[IBIS Ver]   5.0
[Comment Char] |_char
[File name]   k61_120_143wlcsp_full.ibs
[File Rev]   1.1
[Date]   November 08,2016
[Source]   Cadence SpeedXP Suite XtractIM 13.0.2.01241
[Notes]   IBIS model for K61 microprocessor covers 1.71 - 3.6V range
[Disclaimer]   The model given below represents 143WLCSP package on K61 family.
[Copyright]   Copyright, NXP Semiconductors, 2016
|  Component K61
[Component]   K61
[Manufacturer]  NXP Semiconductors
[Package]
|   typ   min   max
R_pkg   0.30362   0.061464   1.7211
L_pkg   1.444e-9   5.12e-10   8.838e-9
C_pkg   1.994e-13   4.495e-14   3.303e-13
[Pin]   Signal_name   model_name   R_pin   L_pin   C_pin
L8   VBAT   POWER
C4   VDD   POWER
E5   VDD   POWER
E7   VDD   POWER
F7   VDD   POWER
G5   VDD   POWER
G7   VDD   POWER
K2   VDD   POWER
L2   VDD   POWER
K11   VDDA   POWER
G9   VOUT33   POWER
K10   VREFH   NC
K9   VREFL   NC
J7   VREFOUT   NC
G8   VREGIN   POWER
L11   DAC0OUT   NC   0.24254   1.143e-9   1.779e-13
K7   DAC1OUT   NC   0.50782   2.109e-9   3.009e-13
L9   EXTAL32   NC   1.7211   8.838e-9   5.089e-14
J10   PGA0DM   NC   0.30343   1.365e-9   2.136e-13
J11   PGA0DP   NC   0.2527   1.165e-9   1.937e-13
J8   PGA1DM   NC   0.42945   1.888e-9   2.645e-13
J9   PGA1DP   NC   0.36354   1.605e-9   2.699e-13
H10   PGA2DM   NC   0.30536   1.372e-9   2.422e-13
H11   PGA2DP   NC   0.23989   1.123e-9   1.938e-13
H8   PGA3DM   NC   0.43162   1.879e-9   2.993e-13
H9   PGA3DP   NC   0.36665   1.611e-9   2.843e-13
K6   PTA0   io_5vtol   0.28835   1.325e-9   2.168e-13
J6   PTA1   io_5vtol   0.3552   1.577e-9   2.756e-13
H5   PTA2   io_5vtol   0.41339   1.804e-9   3.263e-13
J5   PTA3   io_5vtol   0.34455   1.522e-9   2.833e-13
K5   PTA4   io_5vtol   0.28456   1.277e-9   2.245e-13
L5   PTA5   io_5vtol   0.23851   1.144e-9   1.725e-13
L4   PTA12   io_fast_5vtol   0.15229   7.498e-10   1.465e-13
K4   PTA13   io_fast_5vtol   0.21258   9.941e-10   1.823e-13
J4   PTA14   io_fast_5vtol   0.27735   1.255e-9   2.014e-13
L3   PTA15   io_fast_5vtol   0.15747   7.655e-10   1.477e-13
K3   PTA16   io_fast_5vtol   0.22512   1.035e-9   1.845e-13
J3   PTA17   io_fast_5vtol   0.29053   1.305e-9   2.042e-13
L1   PTA18   io_5vtol   0.16163   9.058e-10   5.625e-14
K1   PTA19   io_5vtol   0.14133   7.969e-10   8.082e-14
H4   PTB0   io_5vtol   0.35239   1.586e-9   2.293e-13
H3   PTB1   io_5vtol   0.28722   1.315e-9   2.234e-13
H2   PTB2   io_5vtol   0.22237   1.056e-9   1.795e-13
H1   PTB3   io_5vtol   0.15814   8.112e-10   1.487e-13
G4   PTB4   io_5vtol   0.35452   1.598e-9   2.246e-13
G3   PTB5   io_5vtol   0.28978   1.342e-9   2.086e-13
G2   PTB6   io_5vtol   0.22499   1.085e-9   1.769e-13
G1   PTB7   io_5vtol   0.16003   8.338e-10   1.531e-13
F4   PTB8   io_5vtol   0.35932   1.606e-9   2.315e-13
F3   PTB9   io_5vtol   0.2942   1.36e-9   2.185e-13
F2   PTB10   io_5vtol   0.22996   1.114e-9   1.808e-13
F1   PTB11   io_5vtol   0.16338   8.543e-10   1.457e-13
E1   PTB16   io_5vtol   0.14911   8.121e-10   1.352e-13
E2   PTB17   io_5vtol   0.22144   1.092e-9   1.78e-13
E3   PTB18   io_5vtol   0.28055   1.312e-9   2.128e-13
E4   PTB19   io_5vtol   0.34089   1.552e-9   2.224e-13
D1   PTB20   io_5vtol   0.14359   8.059e-10   1.334e-13
D2   PTB21   io_5vtol   0.2299   1.145e-9   1.782e-13
D5   PTB22   io_5vtol   0.45546   2.026e-9   2.84e-13
D4   PTB23   io_5vtol   0.39466   1.788e-9   2.702e-13
D3   PTC0   io_5vtol   0.30397   1.434e-9   2.149e-13
C1   PTC1   io_5vtol   0.16946   9.36e-10   1.481e-13
C2   PTC2   io_5vtol   0.23273   1.178e-9   1.658e-13
B1   PTC3   io_5vtol   0.15845   9.085e-10   1.371e-13
A3   PTC4   io_5vtol   0.28206   1.417e-9   1.747e-13
B4   PTC5   io_5vtol   0.34473   1.619e-9   2.528e-13
C5   PTC6   io_5vtol   0.43078   1.931e-9   3.218e-13
B5   PTC7   io_5vtol   0.36384   1.676e-9   2.838e-13
A4   PTC8   io_5vtol   0.24808   1.227e-9   2.351e-13
C6   PTC9   io_5vtol   0.43348   1.943e-9   3.055e-13
D6   PTC10   io_5vtol   0.51226   2.248e-9   3.208e-13
A5   PTC11   io_5vtol   0.19355   1.004e-9   1.831e-13
D7   PTC12   io_5vtol   0.42933   1.907e-9   2.765e-13
B6   PTC13   io_5vtol   0.26312   1.265e-9   2.118e-13
C7   PTC14   io_5vtol   0.34241   1.568e-9   2.231e-13
A6   PTC15   io_5vtol   0.16255   8.793e-10   1.509e-13
A7   PTC16   io_5vtol   0.11669   6.909e-10   1.249e-13
B7   PTC17   io_5vtol   0.20702   1.04e-9   1.686e-13
C8   PTC18   io_5vtol   0.26178   1.253e-9   2.001e-13
D8   PTC19   io_5vtol   0.34858   1.589e-9   2.361e-13
B8   PTD0   io_5vtol   0.18881   9.722e-10   1.691e-13
A8   PTD1   io_5vtol   0.11932   7.15e-10   1.257e-13
D9   PTD2   io_5vtol   0.31758   1.477e-9   2.149e-13
C9   PTD3   io_5vtol   0.24617   1.194e-9   1.972e-13
B9   PTD4   io_5vtol   0.17456   9.26e-10   1.545e-13
A9   PTD5   io_5vtol   0.11421   7.019e-10   1.241e-13
B10   PTD6   io_5vtol   0.20692   1.075e-9   1.523e-13
A10   PTD7   io_5vtol   0.061464   5.12e-10   4.495e-14
A11   PTE0   io_5vtol   0.23356   1.226e-9   1.66e-13
C10   PTE1   io_5vtol   0.35054   1.657e-9   2.021e-13
B11   PTE2   io_5vtol   0.24347   1.247e-9   1.579e-13
D10   PTE3   io_5vtol   0.37498   1.744e-9   1.98e-13
C11   PTE4   io_5vtol   0.2325   1.166e-9   1.648e-13
D11   PTE5   io_5vtol   0.23202   1.149e-9   1.726e-13
E9   PTE6   io_5vtol   0.37777   1.714e-9   2.089e-13
E10   PTE7   io_5vtol   0.29186   1.374e-9   1.838e-13
E11   PTE8   io_5vtol   0.22559   1.11e-9   1.778e-13
F8   PTE9   io_5vtol   0.42471   1.869e-9   2.543e-13
F9   PTE10   io_5vtol   0.35943   1.615e-9   2.414e-13
F10   PTE11   io_5vtol   0.29447   1.361e-9   2.086e-13
F11   PTE12   io_5vtol   0.2305   1.117e-9   1.676e-13
L7   PTE24   io_5vtol   0.26232   1.201e-9   2.068e-13
H7   PTE25   io_5vtol   0.4379   1.885e-9   3.303e-13
H6   PTE26   io_5vtol   0.42682   1.834e-9   3.233e-13
L6   PTE27   io_5vtol   0.2373   1.097e-9   2.157e-13
J1   RESETB   NC   0.27914   1.507e-9   6.068e-14
M11   TAMPER0   io_3v   0.18122   9.172e-10   1.558e-13
M10   TAMPER1   io_3v   0.22456   1.074e-9   1.988e-13
M9   TAMPER2   io_3v_trig   0.26705   1.236e-9   2.327e-13
M8   TAMPER3   io_3v   0.31262   1.433e-9   2.187e-13
G10   USB0DM   NC   0.29042   1.331e-9   2.03e-13
G11   USB0DP   NC   0.22626   1.077e-9   1.834e-13
L10   XTAL32   NC   1.4851   7.632e-9   6.574e-14
E6   VSS   GND
E8   VSS   GND
F5   VSS   GND
G6   VSS   GND
J2   VSS   GND
K8   VSSA   GND
|End [Component]
[Component] io65u65dgo6m3v
|   Component io65u65dgo6m3v
| This component was characterised for following simulation conditions:
| Temperature:
|   - Typ: 25.0C,   - Min: 125.0C,   - Max: -40.0C
| External (pad) voltage:
|   - Typ: 3.3V,   - Min: 1.71V,   - Max: 3.6V
| Internal (core) voltage:
|   - Typ: 3.3V,   - Min: 1.71V,   - Max: 3.6V
[Manufacturer] Freescale Semiconductor
[Package]
| variable   typ   min   max
R_pkg   0.2240   0.2240   0.2240
L_pkg   8.5100nH   8.5100nH   8.5100nH
C_pkg   0.2740pF   0.2740pF   0.2740pF
[Pin]  signal_name   model_name   R_pin   L_pin   C_pin
fpad   pad   io_3v_trig
pad   pad   io_3v
vdd3v  vdd3v   POWER
vss3v  vss3v   GND
|obe   obe   dummy
|do   do   dummy
[Model Selector] io_3v_trig
io_3v_trig_dse1_sre0   io with trigger, full drive mode without slew rate
io_3v_trig_dse1_sre1   io with trigger, full drive mode with slew rate
io_3v_trig_dse0_sre0   io with trigger, low drive mode without slew rate
io_3v_trig_dse0_sre1   io with trigger, low drive mode with slew rate
[Model Selector] io_3v
io_3v_dse1_sre0   io, full drive mode without slew rate
io_3v_dse1_sre1   io, full drive mode with slew rate
io_3v_dse0_sre0   io, low drive mode without slew rate
io_3v_dse0_sre1   io, low drive mode with slew rate
[Component] io80u65dgo6m5vtol
|   Component io80u65dgo6m5vtol
| This component was characterised for following simulation conditions:
| Spice Models:
|  - Typ Condition
|   /proj/tec16/analog/modules/IO_C90/io80u65dgo4m5vtol/users/antony/ibis/io80u/6m1t/cmos090sgtfs_typ.model
|  - Min Condition
|   /proj/tec16/analog/modules/IO_C90/io80u65dgo4m5vtol/users/antony/ibis/io80u/6m1t/cmos090sgtfs_wcs.model
|  - Max Condition
|   /proj/tec16/analog/modules/IO_C90/io80u65dgo4m5vtol/users/antony/ibis/io80u/6m1t/cmos090sgtfs_bcs.model
| Spice  Netlist:
|  - Typ Condition
|   /proj/tec16/analog/modules/IO_C90/io80u65dgo4m5vtol/users/antony/ibis/io80u/6m1t/io.ckt
|  - Min Condition
|   /proj/tec16/analog/modules/IO_C90/io80u65dgo4m5vtol/users/antony/ibis/io80u/6m1t/io.ckt
|  - Max Condition
|   /proj/tec16/analog/modules/IO_C90/io80u65dgo4m5vtol/users/antony/ibis/io80u/6m1t/io.ckt
| Temperature:
|   - Typ: 25.0C,   - Min: 125.0C,   - Max: -40.0C
| External (pad) voltage:
|   - Typ: 3.3V,   - Min: 1.71V,   - Max: 3.6V
| Internal (core) voltage:
|   - Typ: 1.2V,   - Min: 1.08V,   - Max: 1.32V
[Manufacturer] Freescale Semiconductor
[Package]
| variable   typ   min   max
R_pkg   0.2240   0.2240   0.2240
L_pkg   8.5100nH   8.5100nH   8.5100nH
C_pkg   0.2740pF   0.2740pF   0.2740pF
[Pin]  signal_name   model_name   R_pin   L_pin   C_pin
fpad   pad   io_fast_5vtol
pad   pad   io_5vtol
|vsslv vsslv   iGND
|vddlv vddlv   iPOWER
vdd3v  vdd3v   POWER
vss3v  vss3v   GND
|obe   obe   dummy
|do   do   dummy
[Model Selector] io_fast_5vtol
io_fast_5vtol_dse1_sre0   fast io, full drive mode without slew rate
io_fast_5vtol_dse1_sre1   fast io, full drive mode with slew rate
io_fast_5vtol_dse0_sre0   fast io, low drive mode without slew rate
io_fast_5vtol_dse0_sre1   fast io, low drive mode with slew rate
[Model Selector] io_5vtol
io_5vtol_dse1_sre0   io, full drive mode without slew rate
io_5vtol_dse1_sre1   io, full drive mode with slew rate
io_5vtol_dse0_sre0   io, low drive mode without slew rate
io_5vtol_dse0_sre1   io, low drive mode with slew rate
| Models and submodels in the file (16): io_3v_trig_dse1_sre0 (I/O), io_3v_dse1_sre0 (I/O), io_3v_trig_dse1_sre1 (I/O), io_3v_dse1_sre1 (I/O), io_3v_trig_dse0_sre0 (I/O), io_3v_dse0_sre0 (I/O), io_3v_trig_dse0_sre1 (I/O), io_3v_dse0_sre1 (I/O), io_fast_5vtol_dse1_sre0 (I/O), io_5vtol_dse1_sre0 (I/O), io_fast_5vtol_dse1_sre1 (I/O), io_5vtol_dse1_sre1 (I/O), io_fast_5vtol_dse0_sre0 (I/O), io_5vtol_dse0_sre0 (I/O), io_fast_5vtol_dse0_sre1 (I/O), io_5vtol_dse0_sre1 (I/O)
